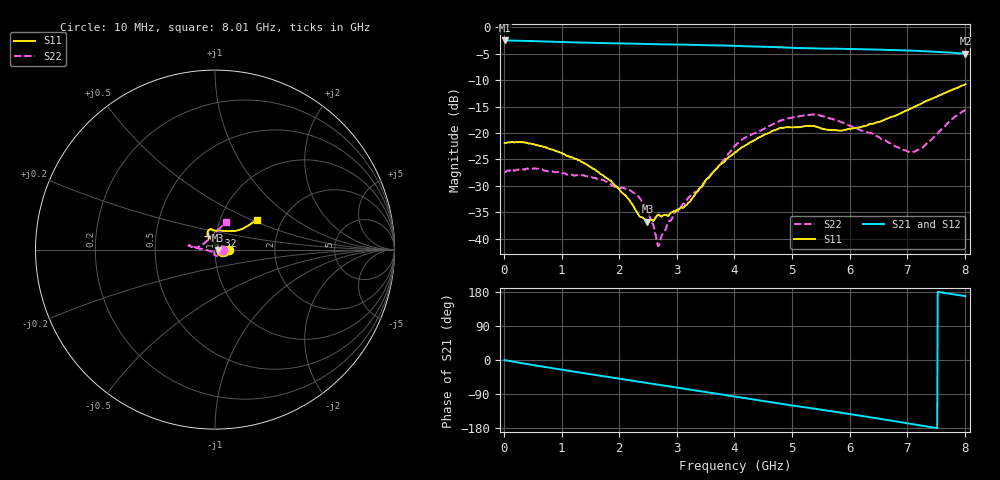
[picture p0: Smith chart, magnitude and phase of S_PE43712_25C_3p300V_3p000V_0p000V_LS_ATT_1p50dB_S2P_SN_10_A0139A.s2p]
! DEVICE ID: PE43712
! File Path: z:\PE43713\PE43713_CHAR_NOM_04292014\AMB\3p300\LS_ATT_1p50dB\PE43713_AMB_3p300V_3p000V_0p000V_LS_ATT_1p50dB_S2P_SN_10_A0139A.s2p
! Serial: 10
! Lot: A0139A
! Temp: 25C
! VDD: 3.300
! VSS: 0.000
! Control_Hi: 3.000
! Control_Lo: 0.000
! Attenuation Step: 1.50dB
! Port 1: RF1
! Port 2: RF2
! ThroughPath:1-2
! IDD: 0.0001468835
! ISS: -1.021e-007
#  Hz  S  RI  R  50
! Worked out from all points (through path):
!   801 points, 10 MHz to 8.01 GHz, reference 50 ohm
!   highest |S21| = -2.52 dB at 10 MHz (marker M1); lowest = -5.0 dB at 8.01 GHz (marker M2)
!   group delay of S21, straight-line fit = 65.6 ps
!   lowest |S11| = -36.8 dB at 2.49 GHz (marker M3), VSWR 1.03, Z = 51.4 - j0.392 ohm
!   |S11| at or under -10 dB: start of sweep to end of sweep
!   |S22| runs from -41.4 to -15.7 dB; largest |S21 - S12| = 0.0022
!   S11 on the Smith chart (normalised r, x): 10 MHz: 1.18, -0.00; 4.32 GHz: 0.92, +0.14; 8.01 GHz: 1.50, +0.54
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1e7  0.0806 -0.00046  0.7478 -0.00405  0.7476 -0.0041  0.0428 -0.000513
3.6e8  0.079 -0.0191  0.7298 -0.1233  0.7317 -0.1228  0.0422 -0.0151
6.8e8  0.0676 -0.0302  0.6973 -0.2238  0.6969 -0.2236  0.0371 -0.0247
1.35e9  0.0379 -0.0372  0.5924 -0.399  0.5921 -0.3988  0.0165 -0.0362
1.84e9  0.0225 -0.0278  0.4941 -0.5018  0.494 -0.5015  0.00464 -0.0328
2.21e9  0.0141 -0.0165  0.4085 -0.5659  0.4086 -0.5656  -0.00423 -0.0279
2.35e9  0.0132 -0.0098  0.3738 -0.5864  0.374 -0.5862  -0.00417 -0.0241
2.49e9  0.014 -0.00381  0.3381 -0.6041  0.3381 -0.6041  -0.00507 -0.0178
2.68e9  0.0156 0.00664  0.2904 -0.6243  0.2906 -0.6242  -0.00235 -0.0082
2.96e9  0.00947 0.0155  0.215 -0.6511  0.2152 -0.6511  -0.0116 -0.0135
3.14e9  0.00443 0.0199  0.1648 -0.6625  0.165 -0.6625  -0.0188 -0.0105
3.41e9  -0.000636 0.0305  0.0892 -0.6713  0.0894 -0.6712  -0.0286 -0.00793
3.71e9  -0.00873 0.0466  0.0066 -0.6707  0.0065 -0.6709  -0.0473 -0.00312
4.01e9  -0.0226 0.0612  -0.0771 -0.6607  -0.0767 -0.6606  -0.0754 0.00393
4.32e9  -0.0379 0.0752  -0.1574 -0.6366  -0.1573 -0.6369  -0.0978 0.00877
4.8e9  -0.0399 0.1042  -0.2743 -0.5829  -0.2737 -0.583  -0.1299 0.0148
5.35e9  -0.0242 0.1138  -0.3841 -0.4983  -0.384 -0.4978  -0.1476 0.0233
5.86e9  0.0113 0.1047  -0.4734 -0.407  -0.4723 -0.407  -0.1252 0.0166
6.68e9  0.0927 0.103  -0.5674 -0.2181  -0.5672 -0.2178  -0.078 0.0215
6.92e9  0.1169 0.1046  -0.5826 -0.1572  -0.5822 -0.1572  -0.059 0.0358
7.15e9  0.1401 0.1114  -0.5897 -0.097  -0.5889 -0.0968  -0.0367 0.0569
8.01e9  0.2349 0.166  -0.5499 0.1122  -0.5484 0.1112  0.06 0.1536
